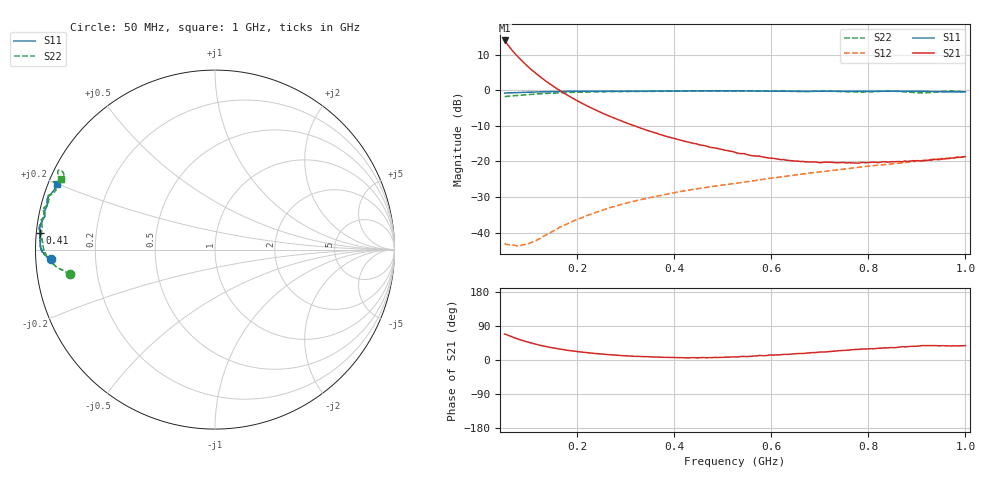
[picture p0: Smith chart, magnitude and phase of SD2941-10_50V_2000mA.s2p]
!Agilent Technologies,E8358A,US42080673,A.04.86
!Agilent E8358A: A.04.86
!Date: Friday, June 09, 2006 14:42:18
!Correction: S11(Full 2 Port SOLT,1,2) S21(Full 2 Port SOLT,1,2) S12(Full 2 Port SOLT,1,2) S22(Full 2 Port SOLT,1,2)
!S2P File: Measurements: S11, S21, S12, S22:
# Hz S  MA  R 50
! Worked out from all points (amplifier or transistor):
!   191 points, 50 MHz to 1 GHz, reference 50 ohm
!   highest |S21| = 14.0 dB at 50 MHz (marker M1)
!   |S21| within 3 dB of that: start of sweep to 66.98 MHz
!   unconditionally stable (mu >= 1): 776.8 MHz to 791.9 MHz; 885.8 MHz to 955.6 MHz; 992.8 MHz to end of sweep
!   at 205 MHz: K = 0.44, MSG = 16.4 dB, |S12| = -36.0 dB
!   at 525 MHz: K = 0.34, MSG = 4.4 dB, |S12| = -26.2 dB
!   at 1 GHz: K = 1.09, MAG = -1.8 dB, |S12| = -18.6 dB
!   S11 on the Smith chart (normalised r, x): 50 MHz: 0.04, -0.03; 410 MHz: 0.01, +0.05; 1 GHz: 0.02, +0.20
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5e7  0.9148 -176.8  5.036 68.8  0.007025 16.0  0.8179 -170.4
5.5e7  0.9218 -176.8  4.508 66.2  0.006791 19.3  0.8253 -170.7
6e7  0.9229 -177.0  4.07 63.6  0.006721 20.7  0.8285 -171.0
6.5e7  0.9234 -177.0  3.695 61.0  0.006754 23.4  0.8358 -171.2
7.5e7  0.9279 -177.3  3.087 56.5  0.006555 30.0  0.8449 -171.9
8e7  0.934 -177.3  2.843 54.3  0.006446 34.5  0.8537 -172.1
9e7  0.9382 -177.6  2.431 50.2  0.006779 40.3  0.8634 -172.5
1.05e8  0.9457 -178.1  1.959 44.8  0.007255 50.1  0.8801 -173.3
1.25e8  0.9532 -178.5  1.523 38.3  0.008369 61.7  0.8973 -174.4
1.45e8  0.9591 -179.1  1.21 33.0  0.01008 68.7  0.9123 -175.4
1.75e8  0.9669 -179.9  0.8927 26.5  0.01289 75.3  0.9305 -176.9
2.1e8  0.9708 179.3  0.6553 20.7  0.01629 77.6  0.9471 -178.7
2.8e8  0.9738 177.3  0.3962 12.4  0.02369 79.2  0.961 177.8
3.7e8  0.9784 175.7  0.2393 7.5  0.03316 78.1  0.9716 174.1
4.1e8  0.9786 174.5  0.2021 6.0  0.03755 76.9  0.9725 172.2
5.25e8  0.9818 172.1  0.1346 8.0  0.04919 74.3  0.9722 168.7
6.85e8  0.9704 168.1  0.09867 19.5  0.06953 69.9  0.9708 162.9
7.85e8  0.9669 165.4  0.09687 28.6  0.08363 66.7  0.9468 159.4
8.45e8  0.9736 163.7  0.09897 32.8  0.09187 65.0  0.9763 157.3
8.95e8  0.9747 162.3  0.1024 36.1  0.1003 63.5  0.9307 156.9
9.6e8  0.9566 159.7  0.1093 37.3  0.111 60.9  0.9726 152.8
1e9  0.9548 157.5  0.1176 38.1  0.1171 57.3  0.9416 155.3
